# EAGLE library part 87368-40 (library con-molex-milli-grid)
RECEPTACAL
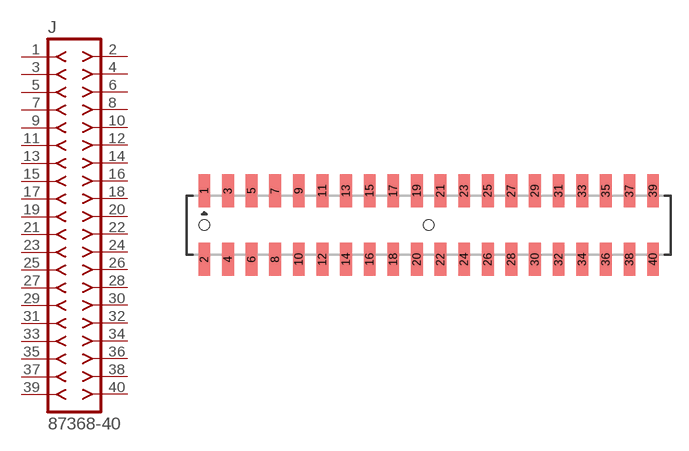
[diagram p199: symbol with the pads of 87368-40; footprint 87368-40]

Designator prefix J

## 87368-40  [87368-40]
1  1  pas
2  2  pas
3  3  pas
4  4  pas
5  5  pas
6  6  pas
7  7  pas
8  8  pas
9  9  pas
10  10  pas
11  11  pas
12  12  pas
13  13  pas
14  14  pas
15  15  pas
16  16  pas
17  17  pas
18  18  pas
19  19  pas
20  20  pas
21  21  pas
22  22  pas
23  23  pas
24  24  pas
25  25  pas
26  26  pas
27  27  pas
28  28  pas
29  29  pas
30  30  pas
31  31  pas
32  32  pas
33  33  pas
34  34  pas
35  35  pas
36  36  pas
37  37  pas
38  38  pas
39  39  pas
40  40  pas

## Footprint 87368-40 (pad centres in mm)
RECEPTACAL SMD Dual Row, Side Entry
smd 1 x 2.8: 1 -19,2.9; 2 -19,-2.9; 3 -17,2.9; 4 -17,-2.9; 5 -15,2.9; 6 -15,-2.9; 7 -13,2.9; 8 -13,-2.9; 9 -11,2.9; 10 -11,-2.9; 11 -9,2.9; 12 -9,-2.9; 13 -7,2.9; 14 -7,-2.9; 15 -5,2.9; 16 -5,-2.9; 17 -3,2.9; 18 -3,-2.9; 19 -1,2.9; 20 -1,-2.9; 21 1,2.9; 22 1,-2.9; 23 3,2.9; 24 3,-2.9; 25 5,2.9; 26 5,-2.9; 27 7,2.9; 28 7,-2.9; 29 9,2.9; 30 9,-2.9; 31 11,2.9; 32 11,-2.9; 33 13,2.9; 34 13,-2.9; 35 15,2.9; 36 15,-2.9; 37 17,2.9; 38 17,-2.9; 39 19,2.9; 40 19,-2.9
hole 0.914 at -19,0
hole 0.914 at 0,0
